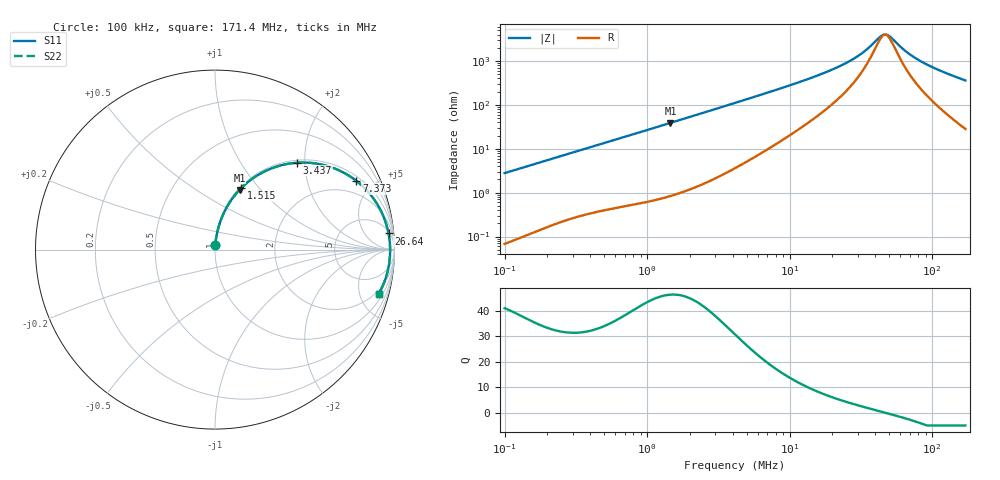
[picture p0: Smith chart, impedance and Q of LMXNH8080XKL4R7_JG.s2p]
! LMXNH8080XKL4R7_JG  S-PARAMETER MODEL  ( General Type )
! Model Generated by TAIYO YUDEN Corporation (https://www.yuden.co.jp/en/)
! Version 1.0
! TAIYO YUDEN Control No. 191025NI43SB-FBB
! Copyright(c) 2019 TAIYO YUDEN CO.,LTD. All Rights Reserved.
! Product Description (link to TY-COMPAS)
! https://ds.yuden.co.jp/TYCOMPAS/or/detail?pn=LMXNH8080XKL4R7MJG&u=M
! Products Name : Inductors
! Characteristics :
!  Inductance : 4.7 uH , SRF(min) : 40 MHz , DC Resistance(max) : 0.0286 Ohm
!  Rated Current : Saturation :3600 mA , Temp Rise : 4000 mA (40 degC)
!  Case Size : 8.0 x 8.0 / 0.315 x 0.315 [mm/inch] , Thickness : 3 / 0.118 [mm/inch]
!  (Conditions: Temperature = 25 degC , DC Bias Current/Voltage = 0A / 0V)
! External Node Assignments :
!  1  o---GGG---o  2
! GND o---------o GND
! Frequency Range : 0.1MHz  -  171.398534MHz  [ 402 STEP ]
# MHz S RI R 50
! Freq[MHz].  S11 Real  S11 Imag  S21 Real  S21 Imag  S12 Real  S12 Imag  S22 Real  S22 Imag
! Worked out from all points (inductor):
!   401 points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, 100 kHz to 171.4 MHz, reference 50 ohm
!   read as one part in series: L = 4.42 uH near 103.8 kHz
!   highest Q = 46.3 at 1.46 MHz (marker M1), where L = 4.24 uH
!   self-resonance near 46.82 MHz
!   S11 on the Smith chart (normalised r, x): 100 kHz: 1.00, +0.06; 1.515 MHz: 1.02, +0.81; 3.437 MHz: 1.05, +1.83; 7.373 MHz: 1.21, +4.00; 26.64 MHz: 6, +20; 171.4 MHz: 1.57, -7.18
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0.1  0.00145 0.0278  0.9985 -0.0278  0.9985 -0.0278  0.00145 0.0278
0.348094  0.0118 0.0932  0.9882 -0.0932  0.9882 -0.0932  0.0118 0.0932
0.667839  0.0353 0.1718  0.9647 -0.1718  0.9647 -0.1718  0.0353 0.1718
1.211692  0.0996 0.2886  0.9004 -0.2886  0.9004 -0.2886  0.0996 0.2886
1.459629  0.1365 0.3327  0.8635 -0.3327  0.8635 -0.3327  0.1365 0.3327
1.515  0.1452 0.3417  0.8548 -0.3417  0.8548 -0.3417  0.1452 0.3417
2.239742  0.267 0.431  0.733 -0.431  0.733 -0.431  0.267 0.431
3.436793  0.4581 0.4841  0.5419 -0.4841  0.5419 -0.4841  0.4581 0.4841
4.140031  0.5492 0.4815  0.4508 -0.4815  0.4508 -0.4815  0.5492 0.4815
7.372913  0.7883 0.3826  0.2117 -0.3826  0.2117 -0.3826  0.7883 0.3826
10.11776  0.8703 0.3011  0.1297 -0.3011  0.1297 -0.3011  0.8703 0.3011
14.41119  0.9256 0.2136  0.0744 -0.2136  0.0744 -0.2136  0.9256 0.2136
20.14791  0.954 0.1418  0.046 -0.1418  0.046 -0.1418  0.954 0.1418
26.63823  0.9668 0.0903  0.0332 -0.0903  0.0332 -0.0903  0.9668 0.0903
33.30624  0.9725 0.0531  0.0275 -0.0531  0.0275 -0.0531  0.9725 0.0531
44.03529  0.9756 0.00943  0.0244 -0.00943  0.0244 -0.00943  0.9756 0.00943
46.5646  0.9757 0.000848  0.0243 -0.000848  0.0243 -0.000848  0.9757 0.000848
50.16444  0.9757 -0.0106  0.0243 0.0106  0.0243 0.0106  0.9757 -0.0106
65.10078  0.9735 -0.0516  0.0265 0.0516  0.0265 0.0516  0.9735 -0.0516
81.39662  0.9685 -0.0891  0.0315 0.0891  0.0315 0.0891  0.9685 -0.0891
113.7985  0.953 -0.1529  0.047 0.1529  0.047 0.1529  0.953 -0.1529
171.3985  0.9118 -0.2469  0.0882 0.2469  0.0882 0.2469  0.9118 -0.2469
